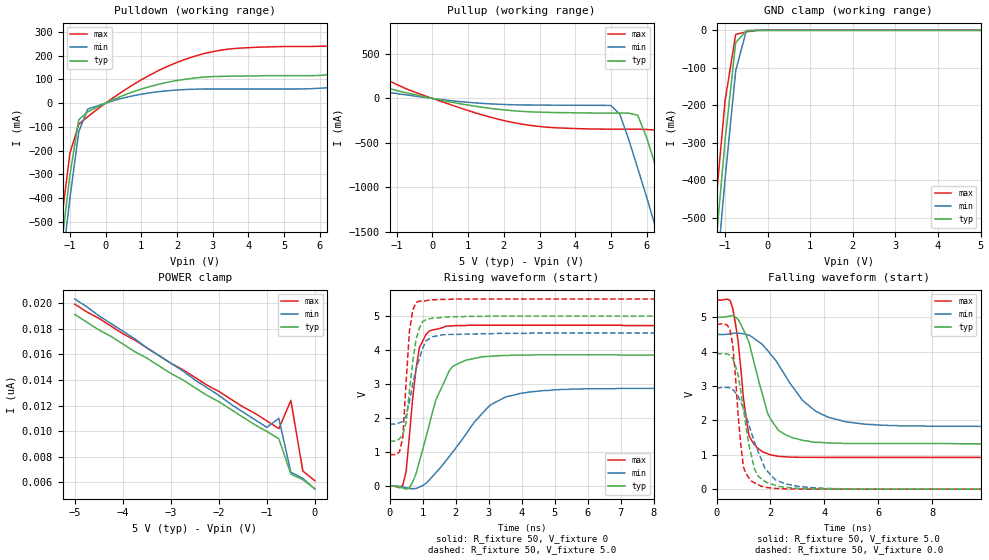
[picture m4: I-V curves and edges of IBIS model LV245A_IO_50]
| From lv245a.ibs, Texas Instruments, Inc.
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|   Model LV245A_IO_50
[Model]   LV245A_IO_50
Model_type  I/O
Polarity   Non-Inverting
Enable   Active-Low
Vinl = 1.5
Vinh = 3.5
Vmeas = 2.5v
Cref = 15pf
| variable   typ   min   max
C_comp   6.0pf   4.5pf   7.5pf
[Temperature Range]   25   85   -40
[Voltage Range]   5.0   4.5   5.5
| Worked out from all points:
|   slope of the pulldown table from 0 to 0.75 V, typ, clamps not added: 16 ohm
|   slope of the pullup table from 0 to 0.75 V, typ, clamps not added: 13 ohm
|   GND clamp passes 1 mA (typ) near -0.46 V on its own axis
|   rising waveform, R_fixture 50, V_fixture 0: 20-80 % time 747ps typ, 1.39ns min, 305ps max; typ from 0 V to 3.85 V
|   falling waveform, R_fixture 50, V_fixture 5.0: 20-80 % time 788ps typ, 1.57ns min, 400ps max; typ from 5 V to 1.32 V
|   rising waveform, R_fixture 50, V_fixture 5.0: 20-80 % time 273ps typ, 404ps min, 178ps max; typ from 1.32 V to 5 V
|   falling waveform, R_fixture 50, V_fixture 0.0: 20-80 % time 512ps typ, 820ps min, 310ps max; typ from 3.94 V to 0 V
[Pulldown]
|   Voltage   I(typ)   I(min)   I(max)
-5V       -5.72A     -5.81A     -5.62A
-1.5V     -947mA     -1.05A     -840mA
-1.25V    -618mA     -720mA     -512mA
-1V       -303mA     -401mA     -211mA
-750mV    -69.4mA    -119mA     -88.1mA
-500mV    -36.3mA    -24.9mA    -57.2mA
500mV     32.8mA     21.9mA     52mA
1.75V     88.6mA     52.6mA     156mA
3V        112mA      59.5mA     217mA
4.25V     115mA      59.7mA     236mA
6.5V      124mA      67.3mA     243mA
10V       155mA      78mA       319mA
[Pullup]
|   Voltage   I(typ)   I(min)   I(max)
-5V       427mA      236mA      797mA
-3.5V     339mA      192mA      620mA
1.5V      -105mA     -57.9mA    -197mA
3V        -154mA     -74.8mA    -316mA
5V        -164mA     -78.5mA    -346mA
5.25V     -164mA     -178mA     -346mA
5.75V     -188mA     -785mA     -346mA
6.25V     -758mA     -1.45A     -356mA
6.5V      -1.09A     -1.78A     -494mA
6.75V     -1.42A     -2.12A     -807mA
7.25V     -2.1A      -2.8A      -1.47A
10V       -5.86A     -6.57A     -5.24A
[GND Clamp]
|   Voltage   I(typ)   I(min)   I(max)
-5V       -5.72A     -5.81A     -5.62A
-1.5V     -945mA     -1.05A     -837mA
-1.25V    -615mA     -718mA     -505mA
-1V       -295mA     -397mA     -188mA
-750mV    -32.5mA    -108mA     -11mA
-500mV    -1.21mA    -785uA     -4.03mA
-250mV    -36nA      -419nA     -157uA
5V        5.52nA     6.8nA      5.11nA
[POWER Clamp]
|   Voltage   I(typ)   I(min)   I(max)
-5V       19.1nA     20.3nA     19.9nA
-4V       16.8nA     17.8nA     17.6nA
-3.75V    16.2nA     17.2nA     17.1nA
-3.5V     15.7nA     16.5nA     16.5nA
-3V       14.5nA     15.3nA     15.3nA
-2.75V    14nA       14.7nA     14.8nA
-1.75V    11.7nA     12.1nA     12.5nA
-1V       9.98nA     10.3nA     10.8nA
-750mV    9.41nA     11nA       10.2nA
-500mV    6.65nA     6.8nA      12.4nA
-250mV    6.22nA     6.32nA     6.89nA
0V        5.52nA     5.48nA     6.14nA
[Ramp]
| variable   typ   min   max
dV/dt_r   2.31E+00/6.67E-10   1.73E+00/1.40E-09   2.84E+00/2.88E-10
dV/dt_f   2.24E+00/7.74E-10   1.63E+00/1.52E-09   2.49E+00/4.56E-10
R_load = 50
[Rising Waveform]
R_fixture = 50
V_fixture = 0
|   Time   V(typ)   V(min)   V(max)
0s        0V         0V         0V
400ps     -62.4mV    -29.4mV    26.6mV
500ps     -95.2mV    -55.4mV    430mV
700ps     123mV      -86.7mV    2.61V
900ps     717mV      -33mV      4.07V
1.4ns     2.53V      388mV      4.61V
1.7ns     3.16V      736mV      4.7V
3.1ns     3.82V      2.41V      4.73V
4.7ns     3.86V      2.81V      4.73V
25ns      3.85V      2.86V      4.72V
[Falling Waveform]
R_fixture = 50
V_fixture = 5.0
V_fixture_min = 4.5
V_fixture_max = 5.5
|   Time   V(typ)   V(min)   V(max)
0s        5V         4.5V       5.5V
600ps     5.05V      4.53V      5.26V
800ps     4.94V      4.54V      4.31V
1ns       4.63V      4.52V      2.65V
1.2ns     4.29V      4.48V      1.57V
2ns       2.05V      3.93V      1V
2.5ns     1.61V      3.37V      945mV
3.7ns     1.36V      2.26V      925mV
5.5ns     1.33V      1.89V      924mV
25ns      1.32V      1.82V      922mV
[Rising Waveform]
R_fixture = 50
V_fixture = 5.0
V_fixture_min = 4.5
V_fixture_max = 5.5
|   Time   V(typ)   V(min)   V(max)
0s        1.32V      1.82V      922mV
300ps     1.39V      1.86V      1.01V
400ps     1.51V      1.9V       1.43V
500ps     1.88V      2.07V      3.07V
600ps     2.81V      2.49V      4.57V
700ps     3.65V      3V         5.17V
900ps     4.64V      3.74V      5.44V
1.1ns     4.89V      4.27V      5.45V
1.8ns     4.97V      4.46V      5.49V
25ns      5V         4.5V       5.5V
[Falling Waveform]
R_fixture = 50
V_fixture = 0.0
|   Time   V(typ)   V(min)   V(max)
0s        3.94V      2.95V      4.8V
500ps     3.9V       2.95V      4.63V
600ps     3.8V       2.9V       4.2V
800ps     3.33V      2.7V       2.18V
1ns       2.33V      2.35V      642mV
1.4ns     617mV      1.38V      189mV
1.7ns     279mV      790mV      76.4mV
2.2ns     108mV      263mV      20.7mV
4ns       4.91mV     25.2mV     2.03mV
25ns      18.9uV     27.7uV     9.69uV
